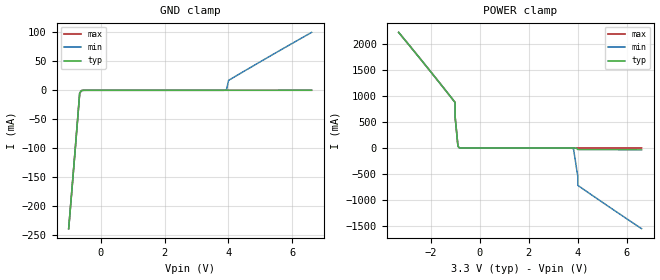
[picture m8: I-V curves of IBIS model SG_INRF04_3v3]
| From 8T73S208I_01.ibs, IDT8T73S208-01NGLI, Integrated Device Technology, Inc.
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[Model] SG_INRF04_3v3
Model_type   Input
Polarity   Non-Inverting
Vinl = 0.8V
Vinh = 2.0V
|   typ   min   max
C_comp   2pF   1.5pF   2.5pF
|   typ   min   max
[Voltage range]   3.3V   3.135V   3.465V
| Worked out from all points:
|   GND clamp passes 1 mA (typ) near -0.60 V on its own axis
|   POWER clamp passes 1 mA (typ) near -0.78 V on its own axis
[GND_clamp]
|Voltage   I (typ)   I (min)   I (max)
-999mV    -239.3mA   -239.3mA   -239.3mA
-826.6mV  -123.8mA   -123.8mA   -123.8mA
-654.2mV  -4.872mA   -4.872mA   -4.872mA
-596.8mV  -528.3uA   -528.3uA   -528.3uA
3.885V    328.8nA    193.5uA    865.9pA
3.943V    3.027uA    1.785mA    5.524nA
4.001V    29.01uA    17.11mA    49.68nA
6.6V      169.8uA    100.1mA    290.7nA
[Power_clamp]
|Voltage   I (typ)   I (min)   I (max)
-3.3V     2.221A     2.221A     2.221A
-1V       874.9mA    874.9mA    874.9mA
-999mV    597.5mA    597.5mA    597.5mA
-884.1mV  34.42mA    34.42mA    34.42mA
-826.6mV  3.732mA    3.732mA    3.732mA
3.77V     -3.951uA   -2.33mA    -6.841nA
3.828V    -36.44uA   -21.48mA   -62.02nA
3.943V    -3.099mA   -373mA     -5.256uA
4V        -28.58mA   -546.1mA   -48.47uA
4.001V    -29.7mA    -717.5mA   -50.38uA
6.6V      -35.17mA   -1.549A    -59.65uA
